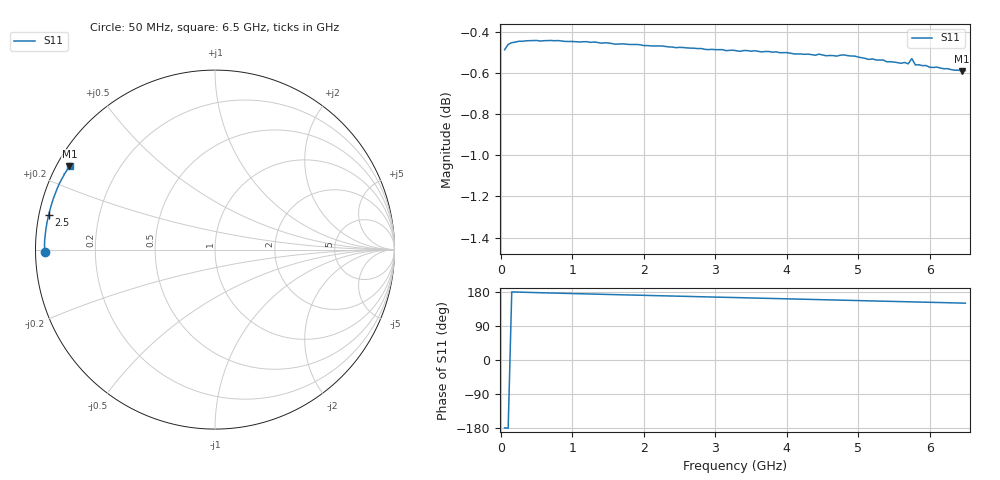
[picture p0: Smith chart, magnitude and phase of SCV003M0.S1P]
! Infineon Technologies  Discrete & RF Semiconductors
! BAR63-02L
! Si PIN Diode in TSLP-2
! IF = 3 mA
! S-Parameters:  March  2002
# GHz  S  MA  R  50
!  f  S11
! GHz  MAG  ANG
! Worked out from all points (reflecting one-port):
!   130 points, 50 MHz to 6.5 GHz, reference 50 ohm
!   lowest |S11| = -0.6 dB at 6.45 GHz (marker M1), VSWR 29.48, Z = 1.82 + j13.3 ohm
!   phase of S11 starts at -179 deg and turns -31 deg over the sweep
!   S11 on the Smith chart (normalised r, x): 50 MHz: 0.03, -0.01; 2.5 GHz: 0.03, +0.10; 6.5 GHz: 0.04, +0.27
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0.05  0.9455 -179.2
0.1  0.9483 -179.9
0.15  0.9492 179.7
0.3  0.95 178.8
0.9  0.9499 175.8
1.1  0.9496 174.9
1.25  0.9494 174.1
1.65  0.9485 172.3
1.7  0.9486 172.0
1.8  0.9483 171.6
2.5  0.9468 168.3
2.9  0.9456 166.5
2.95  0.9457 166.2
3.3  0.9449 164.7
3.95  0.9439 161.6
4.1  0.9433 161.0
4.3  0.9432 160.0
4.4  0.9426 159.6
4.45  0.9432 159.3
4.6  0.9425 158.7
4.8  0.9428 157.7
4.9  0.9422 157.3
5.35  0.9401 155.1
5.7  0.9381 153.6
5.75  0.9408 153.4
5.8  0.9375 153.1
6.45  0.9344 150.2
6.5  0.9345 150.0
